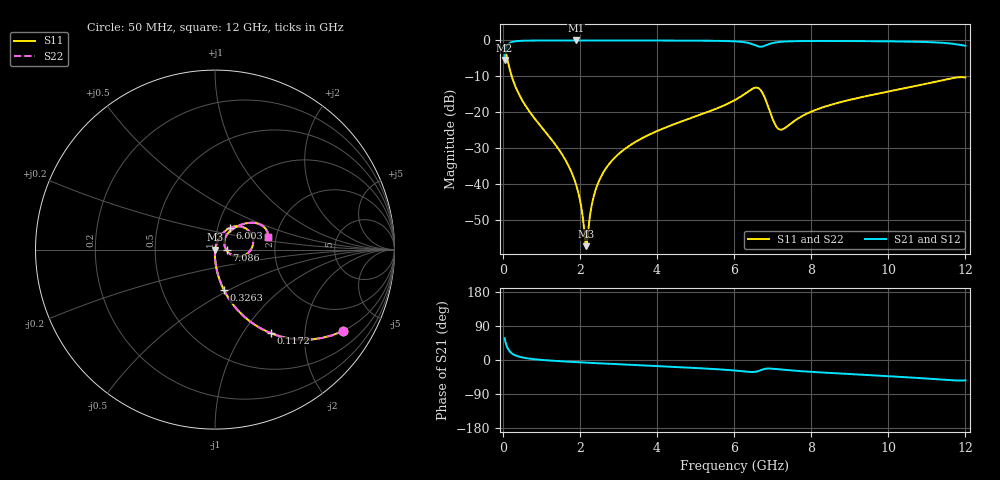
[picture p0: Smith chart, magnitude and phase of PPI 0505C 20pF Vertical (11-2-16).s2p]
# GHz S MA R 50
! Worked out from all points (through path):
!   1601 points, 50 MHz to 12 GHz, reference 50 ohm
!   highest |S21| = -0.01 dB at 1.902 GHz (marker M1); lowest = -5.5 dB at 50 MHz (marker M2)
!   group delay of S21, straight-line fit = 13.9 ps
!   lowest |S11| = -57.3 dB at 2.164 GHz (marker M3), VSWR 1.00, Z = 50.1 - j0.0264 ohm
!   |S11| at or under -10 dB: 235.1 MHz to end of sweep
!   |S22| runs from -57.3 to -1.5 dB; largest |S21 - S12| = 0
!   S11 on the Smith chart (normalised r, x): 50 MHz: 0.99, -3.16; 117.2 MHz: 0.99, -1.34; 326.3 MHz: 0.99, -0.47; 6.003 GHz: 1.14, +0.28; 7.086 GHz: 1.14, -0.01; 12 GHz: 1.81, +0.29
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0.05  0.8458 -32.4  0.5334 57.6  0.5334 57.6  0.8458 -32.4
0.1172187  0.5592 -56.3  0.8287 33.6  0.8287 33.6  0.5592 -56.3
0.199375  0.3669 -69.1  0.9298 20.9  0.9298 20.9  0.3669 -69.1
0.3263437  0.2311 -77.6  0.9723 12.3  0.9723 12.3  0.2311 -77.6
0.6549687  0.1096 -85.4  0.9931 4.2  0.9931 4.2  0.1096 -85.4
1.566156  0.02461 -91.0  0.9984 -3.7  0.9984 -3.7  0.02461 -91.0
1.90225  0.009883 -88.2  0.9986 -5.6  0.9986 -5.6  0.009883 -88.2
2.044156  0.004583 -79.6  0.9985 -6.4  0.9985 -6.4  0.004583 -79.6
2.126313  0.001956 -53.2  0.9985 -6.8  0.9985 -6.8  0.001956 -53.2
2.163656  0.001365 -11.1  0.9985 -7.0  0.9985 -7.0  0.001365 -11.1
2.387719  0.007574 70.9  0.9984 -8.2  0.9984 -8.2  0.007574 70.9
2.679  0.0166 75.1  0.9982 -9.6  0.9982 -9.6  0.0166 75.1
3.201812  0.0318 74.7  0.9976 -12.2  0.9976 -12.2  0.0318 74.7
4.038312  0.05568 71.5  0.996 -16.2  0.996 -16.2  0.05568 71.5
6.002594  0.1459 55.6  0.9718 -27.6  0.9718 -27.6  0.1459 55.6
6.025  0.1481 55.1  0.9704 -27.8  0.9704 -27.8  0.1481 55.1
6.637437  0.216 10.0  0.8226 -29.0  0.8226 -29.0  0.216 10.0
7.085562  0.0646 -3.5  0.9388 -23.9  0.9388 -23.9  0.0646 -3.5
7.264812  0.05801 24.1  0.9612 -25.7  0.9612 -25.7  0.05801 24.1
8.019156  0.1028 51.3  0.9812 -31.4  0.9812 -31.4  0.1028 51.3
10.01331  0.1947 44.4  0.9708 -42.8  0.9708 -42.8  0.1947 44.4
12  0.3046 13.7  0.8422 -53.8  0.8422 -53.8  0.3046 13.7
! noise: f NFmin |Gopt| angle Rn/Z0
0.05  0.0003856  0.865  1.133  0.000613
1.372  0.003925  0.6699  4.61  0.002283
2.701  0.006565  0.6233  8.624  0.00324
4.031  0.009539  0.6164  12.62  0.004575
5.36  0.01696  0.7  16.83  0.01083
6.682  0.1186  0.9394  21.35  0.4218
8.012  0.03229  0.7599  25.26  0.02598
9.341  0.02824  0.6949  28.9  0.01698
10.67  0.03802  0.7375  32.89  0.0267
12  0.1242  0.9021  37.34  0.2496
